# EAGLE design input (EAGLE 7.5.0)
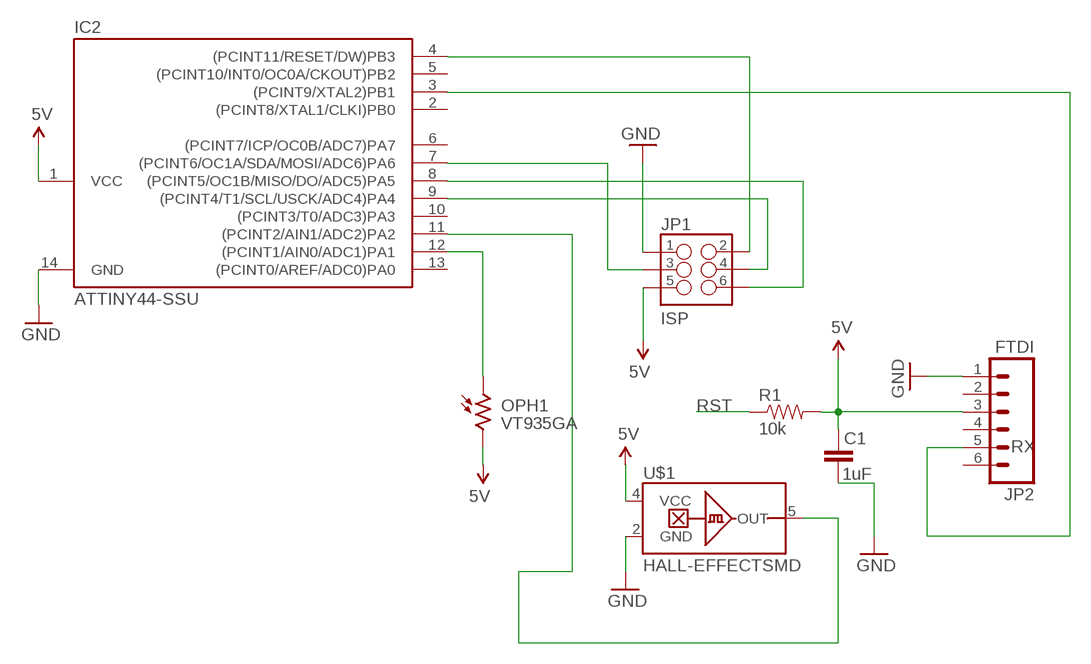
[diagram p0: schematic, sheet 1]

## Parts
C1  1uF  CAP1206  [1206]
IC2  ATTINY44-SSU  [SOIC14]
JP1  ISP  M03X2SMT  [2X3_SMT_POSTS]
JP2  FTDI  M061X06-SMD_EDGE_FEMALE  [1X06-SMD_EDGE]
OPH1  VT935GA  [VT900]
R1  10k  RESISTOR1206  [1206]
U$1  HALL-EFFECTSMD  [SC70]

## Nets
5V: C1.1 IC2.1(VCC) JP1.5 JP2.3 OPH1.2 R1.2 U$1.4(VCC)
GND: C1.2 IC2.14(GND) JP1.1 JP2.1 U$1.2(GND)
N$1: IC2.11((PCINT2/AIN1/ADC2)PA2) U$1.5(OUT)
N$2: IC2.7((PCINT6/OC1A/SDA/MOSI/ADC6)PA6) JP1.3
N$3: IC2.4((PCINT11/RESET/DW)PB3) JP1.2
N$4: IC2.8((PCINT5/OC1B/MISO/DO/ADC5)PA5) JP1.6
N$5: IC2.12((PCINT1/AIN0/ADC1)PA1) OPH1.1
N$6: IC2.3((PCINT9/XTAL2)PB1) JP2.5
RST: R1.1
SCK: IC2.9((PCINT4/T1/SCL/USCK/ADC4)PA4) JP1.4
Unconnected: IC2.2((PCINT8/XTAL1/CLKI)PB0) IC2.5((PCINT10/INT0/OC0A/CKOUT)PB2) IC2.6((PCINT7/ICP/OC0B/ADC7)PA7) IC2.10((PCINT3/T0/ADC3)PA3) IC2.13((PCINT0/AREF/ADC0)PA0) JP2.2 JP2.4 JP2.6

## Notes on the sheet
- RX

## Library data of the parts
C1 = SparkFun-Passives:CAP: Capacitor
IC2 = fab:ATTINY44
JP1 = SparkFun-Connectors:M03X2: 2x3 .1" header. Shrouded, with keying- CONN-10681 SMT- CONN-11415 Pogo pins- HW-11044; PROD_ID: CONN-11415
JP2 = SparkFun-Connectors:M06: Header 6 Standard 6-pin 0.1" header. Use with straight break away headers (SKU : PRT-00116), right angle break away headers (PRT-00553), swiss pins (PRT-00743), machine pins (PRT-00117), and female headers (PRT-00115). Molex polarized connector foot print use with SKU : PRT-08094 with associated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
OPH1 = photo-elements:VT9: Photoconductive Cell VT900 Series
R1 = SparkFun-Passives:RESISTOR: Resistor
U$1 = SparkFun-Sensors:HALL-EFFECT: Hall effect sensor in SC70 package; PROD_ID: IC-09214

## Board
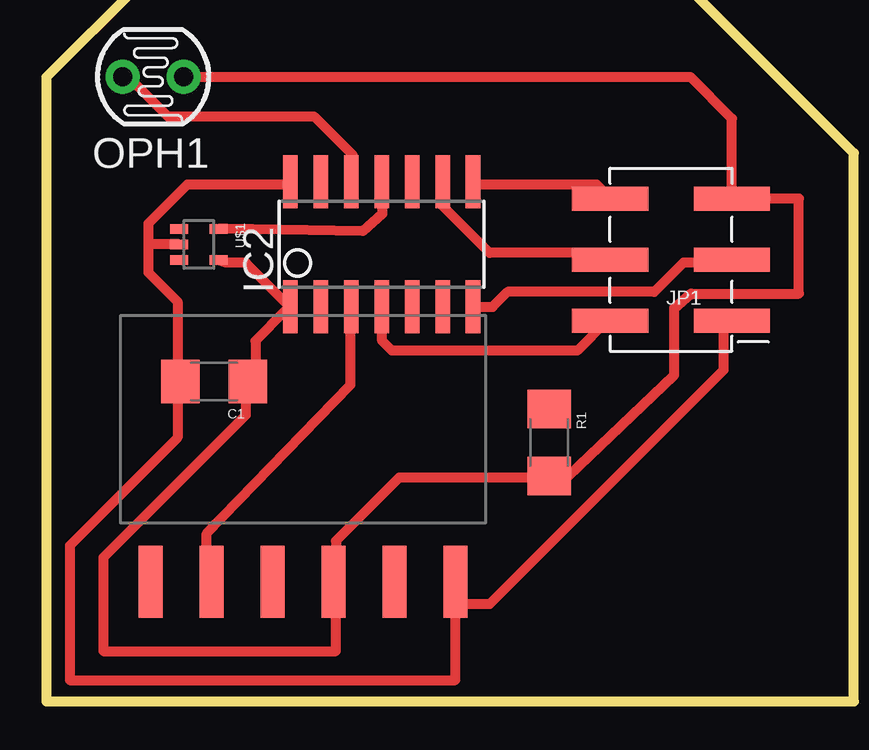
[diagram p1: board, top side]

No outline drawn. Coordinates in mm, seen from the top.
Copper layers (1*16): Top 0.035mm / dielectric 1.5mm / Bottom 0.035mm
Design rules "default *": minimum track width 16mil, minimum drill 24mil, track to track 16mil, track to pad 16mil, pad to pad 16mil, via to via 16mil, smd to smd 16mil, copper to edge 40mil, drill to drill 8mil, minimum pad ring 10mil, minimum via ring 8mil, stop-mask expansion 4mil, vias tented up to drill 0mil, thermal gap 10mil
Milling: 6 lines

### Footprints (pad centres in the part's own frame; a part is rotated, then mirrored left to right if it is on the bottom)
1206 = smd 1.6 x 1.8: 1 -1.4,0; 2 1.4,0
SOIC14 = smd 0.61 x 2.21: 1 -3.81,-2.603; 2 -2.54,-2.603; 3 -1.27,-2.603; 4 0,-2.603; 5 1.27,-2.603; 6 2.54,-2.603; 7 3.81,-2.603; 8 3.81,2.603; 9 2.54,2.603; 10 1.27,2.603; 11 0,2.603; 12 -1.27,2.603; 13 -2.54,2.603; 14 -3.81,2.603
2X3_SMT_POSTS = smd 1 x 3.17: 1 -2.54,-2.54; 2 -2.54,2.54; 3 0,-2.54; 4 0,2.54; 5 2.54,-2.54; 6 2.54,2.54
1X06-SMD_EDGE = smd 1 x 3: 1 0,-0.08; 2 2.54,-0.08; 3 5.08,-0.08; 4 7.62,-0.08; 5 10.16,-0.08; 6 12.7,-0.08
VT900 = drill 0.8 pad 1.4: 1 -1.27,0; 2 1.27,0
SC70 = smd 0.4 x 0.75: 1 -0.65,-0.825; 2 0,-0.825; 3 0.65,-0.825; 4 0.65,0.825; 5 -0.65,0.825

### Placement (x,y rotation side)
C1  7.62,13.34 180 top
IC2  14.61,19.05 0 top
JP1  26.67,18.41 90 top
JP2  17.68,4.91 180 top
OPH1  5.08,26.04 0 top
R1  21.59,10.79 270 top
U$1  6.99,19.05 270 top

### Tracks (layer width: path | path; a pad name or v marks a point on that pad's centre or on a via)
5V
  Top 0.406: U$1.4 8.13,18.29 8.94,18.29 10.57,16.66 IC2.1 10.57,16.26 9.35,15.04 9.35,13.41 C1.1 8.94,13.01 8.94,11.94 3,6 3,2.1 12.7,2.1 12.7,4.99 JP2.3 12.7,5.09 12.7,6.7 15.35,9.35 21.54,9.35 R1.2 22.39,9.39 26.8,13.6 26.8,16.4 27.5,17 32,17 32,20.95 JP1.5 29.21,24.29 27.46,26.04 OPH1.2
GND
  Top 0.406: 4.88,19.05 4.88,19.91 6.5,21.54 10.57,21.54 IC2.14 | 4.88,19.05 4.88,17.88 6.1,16.66 6.1,13.41 C1.2 6.1,13.01 6.1,11 1.6,6.5 1.6,0.9 17.68,0.9 JP2.1 17.88,4.06 19.1,4.06 28.85,13.82 28.85,15.85 JP1.1 | U$1.2 4.88,19.05
N$1
  Top 0.406: U$1.5 8.13,19.71 13.82,19.61 14.63,20.32 14.63,21.54 IC2.11
N$2
  Top 0.406: IC2.7 19.23,16.45 19.85,17.07 25.97,17.07 27.2,18.3 29.09,18.3 JP1.3
N$3
  Top 0.406: IC2.4 14.63,16.26 14.63,15.04 15.04,14.63 22.76,14.63 23.98,15.85 JP1.2
N$4
  Top 0.406: IC2.8 18.69,21.54 23.57,21.54 23.98,21.13 JP1.6
N$5
  Top 0.406: IC2.12 13.41,21.95 13.41,22.76 11.79,24.38 5.69,24.38 4.06,26.01 OPH1.1
N$6
  Top 0.406: 13.41,16.26 IC2.3 13.3,16.28 13.3,13.2 7.32,7.01 7.32,4.06 JP2.5
SCK
  Top 0.406: IC2.9 17.07,21.54 17.07,20.73 19.1,18.69 23.98,18.69 JP1.4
